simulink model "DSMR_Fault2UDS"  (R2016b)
settings: Solver=FixedStepDiscrete  StartTime=0.0  StopTime=10.0  FixedStep=0.02  RelTol=1e-3  EnableMultiTasking=on
undefined symbols (not defined in the file): bin2dec
libraries: simulink x312
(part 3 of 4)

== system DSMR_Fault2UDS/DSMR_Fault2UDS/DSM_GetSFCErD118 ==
  DFC : Inport  OutDataTypeStr=uint8
  DFC_IsoChkLv1_1 : simulink/Logic and Bit Operations/Bitwise Operator  logicop=AND  UseBitMask=on  BitMask=bin2dec('00011000')  BitMaskRealWorld=Stored Integer
  DFC_IsoChkLv1_1_compare : simulink/Logic and Bit Operations/Compare To Constant  relop===  const=24  OutDataTypeStr=boolean
  y : Outport
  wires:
  DFC_IsoChkLv1_1_compare/1 -> y/1
  DFC/1 -> DFC_IsoChkLv1_1/1
  DFC_IsoChkLv1_1/1 -> DFC_IsoChkLv1_1_compare/1

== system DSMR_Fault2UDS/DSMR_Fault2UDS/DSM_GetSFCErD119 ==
  DFC : Inport  OutDataTypeStr=uint8
  DFC_IsoChkLv1_1 : simulink/Logic and Bit Operations/Bitwise Operator  logicop=AND  UseBitMask=on  BitMask=bin2dec('00011000')  BitMaskRealWorld=Stored Integer
  DFC_IsoChkLv1_1_compare : simulink/Logic and Bit Operations/Compare To Constant  relop===  const=24  OutDataTypeStr=boolean
  y : Outport
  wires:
  DFC_IsoChkLv1_1_compare/1 -> y/1
  DFC/1 -> DFC_IsoChkLv1_1/1
  DFC_IsoChkLv1_1/1 -> DFC_IsoChkLv1_1_compare/1

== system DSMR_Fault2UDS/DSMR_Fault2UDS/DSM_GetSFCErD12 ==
  DFC : Inport  OutDataTypeStr=uint8
  DFC_IsoChkLv1_1 : simulink/Logic and Bit Operations/Bitwise Operator  logicop=AND  UseBitMask=on  BitMask=bin2dec('00011000')  BitMaskRealWorld=Stored Integer
  DFC_IsoChkLv1_1_compare : simulink/Logic and Bit Operations/Compare To Constant  relop===  const=24  OutDataTypeStr=boolean
  y : Outport
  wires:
  DFC_IsoChkLv1_1_compare/1 -> y/1
  DFC/1 -> DFC_IsoChkLv1_1/1
  DFC_IsoChkLv1_1/1 -> DFC_IsoChkLv1_1_compare/1

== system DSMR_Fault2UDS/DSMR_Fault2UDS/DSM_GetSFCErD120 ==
  DFC : Inport  OutDataTypeStr=uint8
  DFC_IsoChkLv1_1 : simulink/Logic and Bit Operations/Bitwise Operator  logicop=AND  UseBitMask=on  BitMask=bin2dec('00011000')  BitMaskRealWorld=Stored Integer
  DFC_IsoChkLv1_1_compare : simulink/Logic and Bit Operations/Compare To Constant  relop===  const=24  OutDataTypeStr=boolean
  y : Outport
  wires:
  DFC_IsoChkLv1_1_compare/1 -> y/1
  DFC/1 -> DFC_IsoChkLv1_1/1
  DFC_IsoChkLv1_1/1 -> DFC_IsoChkLv1_1_compare/1

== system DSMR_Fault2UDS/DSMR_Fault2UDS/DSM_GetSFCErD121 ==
  DFC : Inport  OutDataTypeStr=uint8
  DFC_IsoChkLv1_1 : simulink/Logic and Bit Operations/Bitwise Operator  logicop=AND  UseBitMask=on  BitMask=bin2dec('00011000')  BitMaskRealWorld=Stored Integer
  DFC_IsoChkLv1_1_compare : simulink/Logic and Bit Operations/Compare To Constant  relop===  const=24  OutDataTypeStr=boolean
  y : Outport
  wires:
  DFC_IsoChkLv1_1_compare/1 -> y/1
  DFC/1 -> DFC_IsoChkLv1_1/1
  DFC_IsoChkLv1_1/1 -> DFC_IsoChkLv1_1_compare/1

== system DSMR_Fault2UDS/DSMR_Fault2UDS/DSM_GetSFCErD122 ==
  DFC : Inport  OutDataTypeStr=uint8
  DFC_IsoChkLv1_1 : simulink/Logic and Bit Operations/Bitwise Operator  logicop=AND  UseBitMask=on  BitMask=bin2dec('00011000')  BitMaskRealWorld=Stored Integer
  DFC_IsoChkLv1_1_compare : simulink/Logic and Bit Operations/Compare To Constant  relop===  const=24  OutDataTypeStr=boolean
  y : Outport
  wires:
  DFC_IsoChkLv1_1_compare/1 -> y/1
  DFC/1 -> DFC_IsoChkLv1_1/1
  DFC_IsoChkLv1_1/1 -> DFC_IsoChkLv1_1_compare/1

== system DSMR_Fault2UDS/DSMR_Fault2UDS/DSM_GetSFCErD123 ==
  DFC : Inport  OutDataTypeStr=uint8
  DFC_IsoChkLv1_1 : simulink/Logic and Bit Operations/Bitwise Operator  logicop=AND  UseBitMask=on  BitMask=bin2dec('00011000')  BitMaskRealWorld=Stored Integer
  DFC_IsoChkLv1_1_compare : simulink/Logic and Bit Operations/Compare To Constant  relop===  const=24  OutDataTypeStr=boolean
  y : Outport
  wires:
  DFC_IsoChkLv1_1_compare/1 -> y/1
  DFC/1 -> DFC_IsoChkLv1_1/1
  DFC_IsoChkLv1_1/1 -> DFC_IsoChkLv1_1_compare/1

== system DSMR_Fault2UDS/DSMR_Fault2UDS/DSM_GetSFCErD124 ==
  DFC : Inport  OutDataTypeStr=uint8
  DFC_IsoChkLv1_1 : simulink/Logic and Bit Operations/Bitwise Operator  logicop=AND  UseBitMask=on  BitMask=bin2dec('00011000')  BitMaskRealWorld=Stored Integer
  DFC_IsoChkLv1_1_compare : simulink/Logic and Bit Operations/Compare To Constant  relop===  const=24  OutDataTypeStr=boolean
  y : Outport
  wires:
  DFC_IsoChkLv1_1_compare/1 -> y/1
  DFC/1 -> DFC_IsoChkLv1_1/1
  DFC_IsoChkLv1_1/1 -> DFC_IsoChkLv1_1_compare/1

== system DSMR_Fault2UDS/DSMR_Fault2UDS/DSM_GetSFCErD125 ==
  DFC : Inport  OutDataTypeStr=uint8
  DFC_IsoChkLv1_1 : simulink/Logic and Bit Operations/Bitwise Operator  logicop=AND  UseBitMask=on  BitMask=bin2dec('00011000')  BitMaskRealWorld=Stored Integer
  DFC_IsoChkLv1_1_compare : simulink/Logic and Bit Operations/Compare To Constant  relop===  const=24  OutDataTypeStr=boolean
  y : Outport
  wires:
  DFC_IsoChkLv1_1_compare/1 -> y/1
  DFC/1 -> DFC_IsoChkLv1_1/1
  DFC_IsoChkLv1_1/1 -> DFC_IsoChkLv1_1_compare/1

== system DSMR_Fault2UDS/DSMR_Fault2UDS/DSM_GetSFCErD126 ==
  DFC : Inport  OutDataTypeStr=uint8
  DFC_IsoChkLv1_1 : simulink/Logic and Bit Operations/Bitwise Operator  logicop=AND  UseBitMask=on  BitMask=bin2dec('00011000')  BitMaskRealWorld=Stored Integer
  DFC_IsoChkLv1_1_compare : simulink/Logic and Bit Operations/Compare To Constant  relop===  const=24  OutDataTypeStr=boolean
  y : Outport
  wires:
  DFC_IsoChkLv1_1_compare/1 -> y/1
  DFC/1 -> DFC_IsoChkLv1_1/1
  DFC_IsoChkLv1_1/1 -> DFC_IsoChkLv1_1_compare/1

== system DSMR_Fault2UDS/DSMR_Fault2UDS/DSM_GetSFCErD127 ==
  DFC : Inport  OutDataTypeStr=uint8
  DFC_IsoChkLv1_1 : simulink/Logic and Bit Operations/Bitwise Operator  logicop=AND  UseBitMask=on  BitMask=bin2dec('00011000')  BitMaskRealWorld=Stored Integer
  DFC_IsoChkLv1_1_compare : simulink/Logic and Bit Operations/Compare To Constant  relop===  const=24  OutDataTypeStr=boolean
  y : Outport
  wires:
  DFC_IsoChkLv1_1_compare/1 -> y/1
  DFC/1 -> DFC_IsoChkLv1_1/1
  DFC_IsoChkLv1_1/1 -> DFC_IsoChkLv1_1_compare/1

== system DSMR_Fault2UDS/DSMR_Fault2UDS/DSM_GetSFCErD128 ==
  DFC : Inport  OutDataTypeStr=uint8
  DFC_IsoChkLv1_1 : simulink/Logic and Bit Operations/Bitwise Operator  logicop=AND  UseBitMask=on  BitMask=bin2dec('00011000')  BitMaskRealWorld=Stored Integer
  DFC_IsoChkLv1_1_compare : simulink/Logic and Bit Operations/Compare To Constant  relop===  const=24  OutDataTypeStr=boolean
  y : Outport
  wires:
  DFC_IsoChkLv1_1_compare/1 -> y/1
  DFC/1 -> DFC_IsoChkLv1_1/1
  DFC_IsoChkLv1_1/1 -> DFC_IsoChkLv1_1_compare/1

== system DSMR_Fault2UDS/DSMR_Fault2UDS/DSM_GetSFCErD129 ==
  DFC : Inport  OutDataTypeStr=uint8
  DFC_IsoChkLv1_1 : simulink/Logic and Bit Operations/Bitwise Operator  logicop=AND  UseBitMask=on  BitMask=bin2dec('00011000')  BitMaskRealWorld=Stored Integer
  DFC_IsoChkLv1_1_compare : simulink/Logic and Bit Operations/Compare To Constant  relop===  const=24  OutDataTypeStr=boolean
  y : Outport
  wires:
  DFC_IsoChkLv1_1_compare/1 -> y/1
  DFC/1 -> DFC_IsoChkLv1_1/1
  DFC_IsoChkLv1_1/1 -> DFC_IsoChkLv1_1_compare/1

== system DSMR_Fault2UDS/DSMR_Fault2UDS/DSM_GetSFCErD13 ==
  DFC : Inport  OutDataTypeStr=uint8
  DFC_IsoChkLv1_1 : simulink/Logic and Bit Operations/Bitwise Operator  logicop=AND  UseBitMask=on  BitMask=bin2dec('00011000')  BitMaskRealWorld=Stored Integer
  DFC_IsoChkLv1_1_compare : simulink/Logic and Bit Operations/Compare To Constant  relop===  const=24  OutDataTypeStr=boolean
  y : Outport
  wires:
  DFC_IsoChkLv1_1_compare/1 -> y/1
  DFC/1 -> DFC_IsoChkLv1_1/1
  DFC_IsoChkLv1_1/1 -> DFC_IsoChkLv1_1_compare/1

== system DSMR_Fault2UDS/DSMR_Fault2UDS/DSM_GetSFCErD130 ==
  DFC : Inport  OutDataTypeStr=uint8
  DFC_IsoChkLv1_1 : simulink/Logic and Bit Operations/Bitwise Operator  logicop=AND  UseBitMask=on  BitMask=bin2dec('00011000')  BitMaskRealWorld=Stored Integer
  DFC_IsoChkLv1_1_compare : simulink/Logic and Bit Operations/Compare To Constant  relop===  const=24  OutDataTypeStr=boolean
  y : Outport
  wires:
  DFC_IsoChkLv1_1_compare/1 -> y/1
  DFC/1 -> DFC_IsoChkLv1_1/1
  DFC_IsoChkLv1_1/1 -> DFC_IsoChkLv1_1_compare/1

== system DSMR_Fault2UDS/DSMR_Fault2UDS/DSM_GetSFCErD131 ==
  DFC : Inport  OutDataTypeStr=uint8
  DFC_IsoChkLv1_1 : simulink/Logic and Bit Operations/Bitwise Operator  logicop=AND  UseBitMask=on  BitMask=bin2dec('00011000')  BitMaskRealWorld=Stored Integer
  DFC_IsoChkLv1_1_compare : simulink/Logic and Bit Operations/Compare To Constant  relop===  const=24  OutDataTypeStr=boolean
  y : Outport
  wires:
  DFC_IsoChkLv1_1_compare/1 -> y/1
  DFC/1 -> DFC_IsoChkLv1_1/1
  DFC_IsoChkLv1_1/1 -> DFC_IsoChkLv1_1_compare/1

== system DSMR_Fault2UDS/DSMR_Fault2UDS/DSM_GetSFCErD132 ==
  DFC : Inport  OutDataTypeStr=uint8
  DFC_IsoChkLv1_1 : simulink/Logic and Bit Operations/Bitwise Operator  logicop=AND  UseBitMask=on  BitMask=bin2dec('00011000')  BitMaskRealWorld=Stored Integer
  DFC_IsoChkLv1_1_compare : simulink/Logic and Bit Operations/Compare To Constant  relop===  const=24  OutDataTypeStr=boolean
  y : Outport
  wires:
  DFC_IsoChkLv1_1_compare/1 -> y/1
  DFC/1 -> DFC_IsoChkLv1_1/1
  DFC_IsoChkLv1_1/1 -> DFC_IsoChkLv1_1_compare/1

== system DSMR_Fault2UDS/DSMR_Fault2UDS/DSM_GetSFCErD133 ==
  DFC : Inport  OutDataTypeStr=uint8
  DFC_IsoChkLv1_1 : simulink/Logic and Bit Operations/Bitwise Operator  logicop=AND  UseBitMask=on  BitMask=bin2dec('00011000')  BitMaskRealWorld=Stored Integer
  DFC_IsoChkLv1_1_compare : simulink/Logic and Bit Operations/Compare To Constant  relop===  const=24  OutDataTypeStr=boolean
  y : Outport
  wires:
  DFC_IsoChkLv1_1_compare/1 -> y/1
  DFC/1 -> DFC_IsoChkLv1_1/1
  DFC_IsoChkLv1_1/1 -> DFC_IsoChkLv1_1_compare/1

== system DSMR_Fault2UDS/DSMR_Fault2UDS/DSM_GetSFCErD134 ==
  DFC : Inport  OutDataTypeStr=uint8
  DFC_IsoChkLv1_1 : simulink/Logic and Bit Operations/Bitwise Operator  logicop=AND  UseBitMask=on  BitMask=bin2dec('00011000')  BitMaskRealWorld=Stored Integer
  DFC_IsoChkLv1_1_compare : simulink/Logic and Bit Operations/Compare To Constant  relop===  const=24  OutDataTypeStr=boolean
  y : Outport
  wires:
  DFC_IsoChkLv1_1_compare/1 -> y/1
  DFC/1 -> DFC_IsoChkLv1_1/1
  DFC_IsoChkLv1_1/1 -> DFC_IsoChkLv1_1_compare/1

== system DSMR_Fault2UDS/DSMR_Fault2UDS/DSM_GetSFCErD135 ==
  DFC : Inport  OutDataTypeStr=uint8
  DFC_IsoChkLv1_1 : simulink/Logic and Bit Operations/Bitwise Operator  logicop=AND  UseBitMask=on  BitMask=bin2dec('00011000')  BitMaskRealWorld=Stored Integer
  DFC_IsoChkLv1_1_compare : simulink/Logic and Bit Operations/Compare To Constant  relop===  const=24  OutDataTypeStr=boolean
  y : Outport
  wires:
  DFC_IsoChkLv1_1_compare/1 -> y/1
  DFC/1 -> DFC_IsoChkLv1_1/1
  DFC_IsoChkLv1_1/1 -> DFC_IsoChkLv1_1_compare/1

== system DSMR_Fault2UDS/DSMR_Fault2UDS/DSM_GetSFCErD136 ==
  DFC : Inport  OutDataTypeStr=uint8
  DFC_IsoChkLv1_1 : simulink/Logic and Bit Operations/Bitwise Operator  logicop=AND  UseBitMask=on  BitMask=bin2dec('00011000')  BitMaskRealWorld=Stored Integer
  DFC_IsoChkLv1_1_compare : simulink/Logic and Bit Operations/Compare To Constant  relop===  const=24  OutDataTypeStr=boolean
  y : Outport
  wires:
  DFC_IsoChkLv1_1_compare/1 -> y/1
  DFC/1 -> DFC_IsoChkLv1_1/1
  DFC_IsoChkLv1_1/1 -> DFC_IsoChkLv1_1_compare/1

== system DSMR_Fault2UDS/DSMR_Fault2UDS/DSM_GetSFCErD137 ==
  DFC : Inport  OutDataTypeStr=uint8
  DFC_IsoChkLv1_1 : simulink/Logic and Bit Operations/Bitwise Operator  logicop=AND  UseBitMask=on  BitMask=bin2dec('00011000')  BitMaskRealWorld=Stored Integer
  DFC_IsoChkLv1_1_compare : simulink/Logic and Bit Operations/Compare To Constant  relop===  const=24  OutDataTypeStr=boolean
  y : Outport
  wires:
  DFC_IsoChkLv1_1_compare/1 -> y/1
  DFC/1 -> DFC_IsoChkLv1_1/1
  DFC_IsoChkLv1_1/1 -> DFC_IsoChkLv1_1_compare/1

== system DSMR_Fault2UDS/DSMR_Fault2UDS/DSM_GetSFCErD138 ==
  DFC : Inport  OutDataTypeStr=uint8
  DFC_IsoChkLv1_1 : simulink/Logic and Bit Operations/Bitwise Operator  logicop=AND  UseBitMask=on  BitMask=bin2dec('00011000')  BitMaskRealWorld=Stored Integer
  DFC_IsoChkLv1_1_compare : simulink/Logic and Bit Operations/Compare To Constant  relop===  const=24  OutDataTypeStr=boolean
  y : Outport
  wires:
  DFC_IsoChkLv1_1_compare/1 -> y/1
  DFC/1 -> DFC_IsoChkLv1_1/1
  DFC_IsoChkLv1_1/1 -> DFC_IsoChkLv1_1_compare/1

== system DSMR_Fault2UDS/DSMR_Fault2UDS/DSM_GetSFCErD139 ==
  DFC : Inport  OutDataTypeStr=uint8
  DFC_IsoChkLv1_1 : simulink/Logic and Bit Operations/Bitwise Operator  logicop=AND  UseBitMask=on  BitMask=bin2dec('00011000')  BitMaskRealWorld=Stored Integer
  DFC_IsoChkLv1_1_compare : simulink/Logic and Bit Operations/Compare To Constant  relop===  const=24  OutDataTypeStr=boolean
  y : Outport
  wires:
  DFC_IsoChkLv1_1_compare/1 -> y/1
  DFC/1 -> DFC_IsoChkLv1_1/1
  DFC_IsoChkLv1_1/1 -> DFC_IsoChkLv1_1_compare/1

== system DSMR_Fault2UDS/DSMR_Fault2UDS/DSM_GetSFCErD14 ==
  DFC : Inport  OutDataTypeStr=uint8
  DFC_IsoChkLv1_1 : simulink/Logic and Bit Operations/Bitwise Operator  logicop=AND  UseBitMask=on  BitMask=bin2dec('00011000')  BitMaskRealWorld=Stored Integer
  DFC_IsoChkLv1_1_compare : simulink/Logic and Bit Operations/Compare To Constant  relop===  const=24  OutDataTypeStr=boolean
  y : Outport
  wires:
  DFC_IsoChkLv1_1_compare/1 -> y/1
  DFC/1 -> DFC_IsoChkLv1_1/1
  DFC_IsoChkLv1_1/1 -> DFC_IsoChkLv1_1_compare/1

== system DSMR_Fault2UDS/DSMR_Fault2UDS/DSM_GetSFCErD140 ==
  DFC : Inport  OutDataTypeStr=uint8
  DFC_IsoChkLv1_1 : simulink/Logic and Bit Operations/Bitwise Operator  logicop=AND  UseBitMask=on  BitMask=bin2dec('00011000')  BitMaskRealWorld=Stored Integer
  DFC_IsoChkLv1_1_compare : simulink/Logic and Bit Operations/Compare To Constant  relop===  const=24  OutDataTypeStr=boolean
  y : Outport
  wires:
  DFC_IsoChkLv1_1_compare/1 -> y/1
  DFC/1 -> DFC_IsoChkLv1_1/1
  DFC_IsoChkLv1_1/1 -> DFC_IsoChkLv1_1_compare/1

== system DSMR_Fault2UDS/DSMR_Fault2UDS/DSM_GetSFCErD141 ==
  DFC : Inport  OutDataTypeStr=uint8
  DFC_IsoChkLv1_1 : simulink/Logic and Bit Operations/Bitwise Operator  logicop=AND  UseBitMask=on  BitMask=bin2dec('00011000')  BitMaskRealWorld=Stored Integer
  DFC_IsoChkLv1_1_compare : simulink/Logic and Bit Operations/Compare To Constant  relop===  const=24  OutDataTypeStr=boolean
  y : Outport
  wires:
  DFC_IsoChkLv1_1_compare/1 -> y/1
  DFC/1 -> DFC_IsoChkLv1_1/1
  DFC_IsoChkLv1_1/1 -> DFC_IsoChkLv1_1_compare/1

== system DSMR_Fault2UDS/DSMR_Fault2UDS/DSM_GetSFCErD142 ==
  DFC : Inport  OutDataTypeStr=uint8
  DFC_IsoChkLv1_1 : simulink/Logic and Bit Operations/Bitwise Operator  logicop=AND  UseBitMask=on  BitMask=bin2dec('00011000')  BitMaskRealWorld=Stored Integer
  DFC_IsoChkLv1_1_compare : simulink/Logic and Bit Operations/Compare To Constant  relop===  const=24  OutDataTypeStr=boolean
  y : Outport
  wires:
  DFC_IsoChkLv1_1_compare/1 -> y/1
  DFC/1 -> DFC_IsoChkLv1_1/1
  DFC_IsoChkLv1_1/1 -> DFC_IsoChkLv1_1_compare/1

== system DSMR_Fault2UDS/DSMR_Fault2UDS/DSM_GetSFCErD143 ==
  DFC : Inport  OutDataTypeStr=uint8
  DFC_IsoChkLv1_1 : simulink/Logic and Bit Operations/Bitwise Operator  logicop=AND  UseBitMask=on  BitMask=bin2dec('00011000')  BitMaskRealWorld=Stored Integer
  DFC_IsoChkLv1_1_compare : simulink/Logic and Bit Operations/Compare To Constant  relop===  const=24  OutDataTypeStr=boolean
  y : Outport
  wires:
  DFC_IsoChkLv1_1_compare/1 -> y/1
  DFC/1 -> DFC_IsoChkLv1_1/1
  DFC_IsoChkLv1_1/1 -> DFC_IsoChkLv1_1_compare/1

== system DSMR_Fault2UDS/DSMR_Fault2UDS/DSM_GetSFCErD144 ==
  DFC : Inport  OutDataTypeStr=uint8
  DFC_IsoChkLv1_1 : simulink/Logic and Bit Operations/Bitwise Operator  logicop=AND  UseBitMask=on  BitMask=bin2dec('00011000')  BitMaskRealWorld=Stored Integer
  DFC_IsoChkLv1_1_compare : simulink/Logic and Bit Operations/Compare To Constant  relop===  const=24  OutDataTypeStr=boolean
  y : Outport
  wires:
  DFC_IsoChkLv1_1_compare/1 -> y/1
  DFC/1 -> DFC_IsoChkLv1_1/1
  DFC_IsoChkLv1_1/1 -> DFC_IsoChkLv1_1_compare/1

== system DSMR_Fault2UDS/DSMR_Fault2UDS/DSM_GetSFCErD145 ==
  DFC : Inport  OutDataTypeStr=uint8
  DFC_IsoChkLv1_1 : simulink/Logic and Bit Operations/Bitwise Operator  logicop=AND  UseBitMask=on  BitMask=bin2dec('00011000')  BitMaskRealWorld=Stored Integer
  DFC_IsoChkLv1_1_compare : simulink/Logic and Bit Operations/Compare To Constant  relop===  const=24  OutDataTypeStr=boolean
  y : Outport
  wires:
  DFC_IsoChkLv1_1_compare/1 -> y/1
  DFC/1 -> DFC_IsoChkLv1_1/1
  DFC_IsoChkLv1_1/1 -> DFC_IsoChkLv1_1_compare/1

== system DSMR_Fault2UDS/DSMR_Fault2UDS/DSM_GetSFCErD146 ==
  DFC : Inport  OutDataTypeStr=uint8
  DFC_IsoChkLv1_1 : simulink/Logic and Bit Operations/Bitwise Operator  logicop=AND  UseBitMask=on  BitMask=bin2dec('00011000')  BitMaskRealWorld=Stored Integer
  DFC_IsoChkLv1_1_compare : simulink/Logic and Bit Operations/Compare To Constant  relop===  const=24  OutDataTypeStr=boolean
  y : Outport
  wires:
  DFC_IsoChkLv1_1_compare/1 -> y/1
  DFC/1 -> DFC_IsoChkLv1_1/1
  DFC_IsoChkLv1_1/1 -> DFC_IsoChkLv1_1_compare/1

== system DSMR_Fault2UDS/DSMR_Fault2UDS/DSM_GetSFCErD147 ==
  DFC : Inport  OutDataTypeStr=uint8
  DFC_IsoChkLv1_1 : simulink/Logic and Bit Operations/Bitwise Operator  logicop=AND  UseBitMask=on  BitMask=bin2dec('00011000')  BitMaskRealWorld=Stored Integer
  DFC_IsoChkLv1_1_compare : simulink/Logic and Bit Operations/Compare To Constant  relop===  const=24  OutDataTypeStr=boolean
  y : Outport
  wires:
  DFC_IsoChkLv1_1_compare/1 -> y/1
  DFC/1 -> DFC_IsoChkLv1_1/1
  DFC_IsoChkLv1_1/1 -> DFC_IsoChkLv1_1_compare/1

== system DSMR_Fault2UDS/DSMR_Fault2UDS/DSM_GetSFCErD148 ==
  DFC : Inport  OutDataTypeStr=uint8
  DFC_IsoChkLv1_1 : simulink/Logic and Bit Operations/Bitwise Operator  logicop=AND  UseBitMask=on  BitMask=bin2dec('00011000')  BitMaskRealWorld=Stored Integer
  DFC_IsoChkLv1_1_compare : simulink/Logic and Bit Operations/Compare To Constant  relop===  const=24  OutDataTypeStr=boolean
  y : Outport
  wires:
  DFC_IsoChkLv1_1_compare/1 -> y/1
  DFC/1 -> DFC_IsoChkLv1_1/1
  DFC_IsoChkLv1_1/1 -> DFC_IsoChkLv1_1_compare/1

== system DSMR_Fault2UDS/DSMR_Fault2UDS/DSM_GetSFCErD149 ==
  DFC : Inport  OutDataTypeStr=uint8
  DFC_IsoChkLv1_1 : simulink/Logic and Bit Operations/Bitwise Operator  logicop=AND  UseBitMask=on  BitMask=bin2dec('00011000')  BitMaskRealWorld=Stored Integer
  DFC_IsoChkLv1_1_compare : simulink/Logic and Bit Operations/Compare To Constant  relop===  const=24  OutDataTypeStr=boolean
  y : Outport
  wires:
  DFC_IsoChkLv1_1_compare/1 -> y/1
  DFC/1 -> DFC_IsoChkLv1_1/1
  DFC_IsoChkLv1_1/1 -> DFC_IsoChkLv1_1_compare/1

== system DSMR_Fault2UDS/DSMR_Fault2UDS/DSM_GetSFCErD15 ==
  DFC : Inport  OutDataTypeStr=uint8
  DFC_IsoChkLv1_1 : simulink/Logic and Bit Operations/Bitwise Operator  logicop=AND  UseBitMask=on  BitMask=bin2dec('00011000')  BitMaskRealWorld=Stored Integer
  DFC_IsoChkLv1_1_compare : simulink/Logic and Bit Operations/Compare To Constant  relop===  const=24  OutDataTypeStr=boolean
  y : Outport
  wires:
  DFC_IsoChkLv1_1_compare/1 -> y/1
  DFC/1 -> DFC_IsoChkLv1_1/1
  DFC_IsoChkLv1_1/1 -> DFC_IsoChkLv1_1_compare/1

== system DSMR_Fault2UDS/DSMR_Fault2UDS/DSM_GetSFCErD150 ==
  DFC : Inport  OutDataTypeStr=uint8
  DFC_IsoChkLv1_1 : simulink/Logic and Bit Operations/Bitwise Operator  logicop=AND  UseBitMask=on  BitMask=bin2dec('00011000')  BitMaskRealWorld=Stored Integer
  DFC_IsoChkLv1_1_compare : simulink/Logic and Bit Operations/Compare To Constant  relop===  const=24  OutDataTypeStr=boolean
  y : Outport
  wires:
  DFC_IsoChkLv1_1_compare/1 -> y/1
  DFC/1 -> DFC_IsoChkLv1_1/1
  DFC_IsoChkLv1_1/1 -> DFC_IsoChkLv1_1_compare/1

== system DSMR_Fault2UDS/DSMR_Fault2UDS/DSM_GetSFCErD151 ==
  DFC : Inport  OutDataTypeStr=uint8
  DFC_IsoChkLv1_1 : simulink/Logic and Bit Operations/Bitwise Operator  logicop=AND  UseBitMask=on  BitMask=bin2dec('00011000')  BitMaskRealWorld=Stored Integer
  DFC_IsoChkLv1_1_compare : simulink/Logic and Bit Operations/Compare To Constant  relop===  const=24  OutDataTypeStr=boolean
  y : Outport
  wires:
  DFC_IsoChkLv1_1_compare/1 -> y/1
  DFC/1 -> DFC_IsoChkLv1_1/1
  DFC_IsoChkLv1_1/1 -> DFC_IsoChkLv1_1_compare/1

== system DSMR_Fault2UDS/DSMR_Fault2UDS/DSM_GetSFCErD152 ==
  DFC : Inport  OutDataTypeStr=uint8
  DFC_IsoChkLv1_1 : simulink/Logic and Bit Operations/Bitwise Operator  logicop=AND  UseBitMask=on  BitMask=bin2dec('00011000')  BitMaskRealWorld=Stored Integer
  DFC_IsoChkLv1_1_compare : simulink/Logic and Bit Operations/Compare To Constant  relop===  const=24  OutDataTypeStr=boolean
  y : Outport
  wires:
  DFC_IsoChkLv1_1_compare/1 -> y/1
  DFC/1 -> DFC_IsoChkLv1_1/1
  DFC_IsoChkLv1_1/1 -> DFC_IsoChkLv1_1_compare/1

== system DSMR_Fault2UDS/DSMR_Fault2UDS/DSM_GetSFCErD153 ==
  DFC : Inport  OutDataTypeStr=uint8
  DFC_IsoChkLv1_1 : simulink/Logic and Bit Operations/Bitwise Operator  logicop=AND  UseBitMask=on  BitMask=bin2dec('00011000')  BitMaskRealWorld=Stored Integer
  DFC_IsoChkLv1_1_compare : simulink/Logic and Bit Operations/Compare To Constant  relop===  const=24  OutDataTypeStr=boolean
  y : Outport
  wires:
  DFC_IsoChkLv1_1_compare/1 -> y/1
  DFC/1 -> DFC_IsoChkLv1_1/1
  DFC_IsoChkLv1_1/1 -> DFC_IsoChkLv1_1_compare/1

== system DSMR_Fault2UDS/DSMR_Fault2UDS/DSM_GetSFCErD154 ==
  DFC : Inport  OutDataTypeStr=uint8
  DFC_IsoChkLv1_1 : simulink/Logic and Bit Operations/Bitwise Operator  logicop=AND  UseBitMask=on  BitMask=bin2dec('00011000')  BitMaskRealWorld=Stored Integer
  DFC_IsoChkLv1_1_compare : simulink/Logic and Bit Operations/Compare To Constant  relop===  const=24  OutDataTypeStr=boolean
  y : Outport
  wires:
  DFC_IsoChkLv1_1_compare/1 -> y/1
  DFC/1 -> DFC_IsoChkLv1_1/1
  DFC_IsoChkLv1_1/1 -> DFC_IsoChkLv1_1_compare/1

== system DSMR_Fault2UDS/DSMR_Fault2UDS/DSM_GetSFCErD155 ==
  DFC : Inport  OutDataTypeStr=uint8
  DFC_IsoChkLv1_1 : simulink/Logic and Bit Operations/Bitwise Operator  logicop=AND  UseBitMask=on  BitMask=bin2dec('00011000')  BitMaskRealWorld=Stored Integer
  DFC_IsoChkLv1_1_compare : simulink/Logic and Bit Operations/Compare To Constant  relop===  const=24  OutDataTypeStr=boolean
  y : Outport
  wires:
  DFC_IsoChkLv1_1_compare/1 -> y/1
  DFC/1 -> DFC_IsoChkLv1_1/1
  DFC_IsoChkLv1_1/1 -> DFC_IsoChkLv1_1_compare/1

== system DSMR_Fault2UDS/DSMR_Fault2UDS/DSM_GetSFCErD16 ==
  DFC : Inport  OutDataTypeStr=uint8
  DFC_IsoChkLv1_1 : simulink/Logic and Bit Operations/Bitwise Operator  logicop=AND  UseBitMask=on  BitMask=bin2dec('00011000')  BitMaskRealWorld=Stored Integer
  DFC_IsoChkLv1_1_compare : simulink/Logic and Bit Operations/Compare To Constant  relop===  const=24  OutDataTypeStr=boolean
  y : Outport
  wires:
  DFC_IsoChkLv1_1_compare/1 -> y/1
  DFC/1 -> DFC_IsoChkLv1_1/1
  DFC_IsoChkLv1_1/1 -> DFC_IsoChkLv1_1_compare/1

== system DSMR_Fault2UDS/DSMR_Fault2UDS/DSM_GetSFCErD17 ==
  DFC : Inport  OutDataTypeStr=uint8
  DFC_IsoChkLv1_1 : simulink/Logic and Bit Operations/Bitwise Operator  logicop=AND  UseBitMask=on  BitMask=bin2dec('00011000')  BitMaskRealWorld=Stored Integer
  DFC_IsoChkLv1_1_compare : simulink/Logic and Bit Operations/Compare To Constant  relop===  const=24  OutDataTypeStr=boolean
  y : Outport
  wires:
  DFC_IsoChkLv1_1_compare/1 -> y/1
  DFC/1 -> DFC_IsoChkLv1_1/1
  DFC_IsoChkLv1_1/1 -> DFC_IsoChkLv1_1_compare/1

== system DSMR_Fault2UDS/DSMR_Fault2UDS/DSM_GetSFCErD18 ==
  DFC : Inport  OutDataTypeStr=uint8
  DFC_IsoChkLv1_1 : simulink/Logic and Bit Operations/Bitwise Operator  logicop=AND  UseBitMask=on  BitMask=bin2dec('00011000')  BitMaskRealWorld=Stored Integer
  DFC_IsoChkLv1_1_compare : simulink/Logic and Bit Operations/Compare To Constant  relop===  const=24  OutDataTypeStr=boolean
  y : Outport
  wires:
  DFC_IsoChkLv1_1_compare/1 -> y/1
  DFC/1 -> DFC_IsoChkLv1_1/1
  DFC_IsoChkLv1_1/1 -> DFC_IsoChkLv1_1_compare/1

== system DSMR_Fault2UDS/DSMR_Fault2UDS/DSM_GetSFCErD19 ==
  DFC : Inport  OutDataTypeStr=uint8
  DFC_IsoChkLv1_1 : simulink/Logic and Bit Operations/Bitwise Operator  logicop=AND  UseBitMask=on  BitMask=bin2dec('00011000')  BitMaskRealWorld=Stored Integer
  DFC_IsoChkLv1_1_compare : simulink/Logic and Bit Operations/Compare To Constant  relop===  const=24  OutDataTypeStr=boolean
  y : Outport
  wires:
  DFC_IsoChkLv1_1_compare/1 -> y/1
  DFC/1 -> DFC_IsoChkLv1_1/1
  DFC_IsoChkLv1_1/1 -> DFC_IsoChkLv1_1_compare/1

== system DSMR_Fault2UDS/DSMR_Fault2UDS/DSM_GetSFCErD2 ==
  DFC : Inport  OutDataTypeStr=uint8
  DFC_IsoChkLv1_1 : simulink/Logic and Bit Operations/Bitwise Operator  logicop=AND  UseBitMask=on  BitMask=bin2dec('00011000')  BitMaskRealWorld=Stored Integer
  DFC_IsoChkLv1_1_compare : simulink/Logic and Bit Operations/Compare To Constant  relop===  const=24  OutDataTypeStr=boolean
  y : Outport
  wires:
  DFC_IsoChkLv1_1_compare/1 -> y/1
  DFC/1 -> DFC_IsoChkLv1_1/1
  DFC_IsoChkLv1_1/1 -> DFC_IsoChkLv1_1_compare/1

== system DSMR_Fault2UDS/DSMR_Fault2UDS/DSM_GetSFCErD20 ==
  DFC : Inport  OutDataTypeStr=uint8
  DFC_IsoChkLv1_1 : simulink/Logic and Bit Operations/Bitwise Operator  logicop=AND  UseBitMask=on  BitMask=bin2dec('00011000')  BitMaskRealWorld=Stored Integer
  DFC_IsoChkLv1_1_compare : simulink/Logic and Bit Operations/Compare To Constant  relop===  const=24  OutDataTypeStr=boolean
  y : Outport
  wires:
  DFC_IsoChkLv1_1_compare/1 -> y/1
  DFC/1 -> DFC_IsoChkLv1_1/1
  DFC_IsoChkLv1_1/1 -> DFC_IsoChkLv1_1_compare/1

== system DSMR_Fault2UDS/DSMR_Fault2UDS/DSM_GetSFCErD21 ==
  DFC : Inport  OutDataTypeStr=uint8
  DFC_IsoChkLv1_1 : simulink/Logic and Bit Operations/Bitwise Operator  logicop=AND  UseBitMask=on  BitMask=bin2dec('00011000')  BitMaskRealWorld=Stored Integer
  DFC_IsoChkLv1_1_compare : simulink/Logic and Bit Operations/Compare To Constant  relop===  const=24  OutDataTypeStr=boolean
  y : Outport
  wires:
  DFC_IsoChkLv1_1_compare/1 -> y/1
  DFC/1 -> DFC_IsoChkLv1_1/1
  DFC_IsoChkLv1_1/1 -> DFC_IsoChkLv1_1_compare/1

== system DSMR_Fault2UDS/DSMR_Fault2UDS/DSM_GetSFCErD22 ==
  DFC : Inport  OutDataTypeStr=uint8
  DFC_IsoChkLv1_1 : simulink/Logic and Bit Operations/Bitwise Operator  logicop=AND  UseBitMask=on  BitMask=bin2dec('00011000')  BitMaskRealWorld=Stored Integer
  DFC_IsoChkLv1_1_compare : simulink/Logic and Bit Operations/Compare To Constant  relop===  const=24  OutDataTypeStr=boolean
  y : Outport
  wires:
  DFC_IsoChkLv1_1_compare/1 -> y/1
  DFC/1 -> DFC_IsoChkLv1_1/1
  DFC_IsoChkLv1_1/1 -> DFC_IsoChkLv1_1_compare/1

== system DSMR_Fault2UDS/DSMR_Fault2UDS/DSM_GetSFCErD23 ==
  DFC : Inport  OutDataTypeStr=uint8
  DFC_IsoChkLv1_1 : simulink/Logic and Bit Operations/Bitwise Operator  logicop=AND  UseBitMask=on  BitMask=bin2dec('00011000')  BitMaskRealWorld=Stored Integer
  DFC_IsoChkLv1_1_compare : simulink/Logic and Bit Operations/Compare To Constant  relop===  const=24  OutDataTypeStr=boolean
  y : Outport
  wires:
  DFC_IsoChkLv1_1_compare/1 -> y/1
  DFC/1 -> DFC_IsoChkLv1_1/1
  DFC_IsoChkLv1_1/1 -> DFC_IsoChkLv1_1_compare/1

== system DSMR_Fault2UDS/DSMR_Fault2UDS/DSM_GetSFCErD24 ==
  DFC : Inport  OutDataTypeStr=uint8
  DFC_IsoChkLv1_1 : simulink/Logic and Bit Operations/Bitwise Operator  logicop=AND  UseBitMask=on  BitMask=bin2dec('00011000')  BitMaskRealWorld=Stored Integer
  DFC_IsoChkLv1_1_compare : simulink/Logic and Bit Operations/Compare To Constant  relop===  const=24  OutDataTypeStr=boolean
  y : Outport
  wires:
  DFC_IsoChkLv1_1_compare/1 -> y/1
  DFC/1 -> DFC_IsoChkLv1_1/1
  DFC_IsoChkLv1_1/1 -> DFC_IsoChkLv1_1_compare/1

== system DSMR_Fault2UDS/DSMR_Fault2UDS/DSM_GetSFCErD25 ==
  DFC : Inport  OutDataTypeStr=uint8
  DFC_IsoChkLv1_1 : simulink/Logic and Bit Operations/Bitwise Operator  logicop=AND  UseBitMask=on  BitMask=bin2dec('00011000')  BitMaskRealWorld=Stored Integer
  DFC_IsoChkLv1_1_compare : simulink/Logic and Bit Operations/Compare To Constant  relop===  const=24  OutDataTypeStr=boolean
  y : Outport
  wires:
  DFC_IsoChkLv1_1_compare/1 -> y/1
  DFC/1 -> DFC_IsoChkLv1_1/1
  DFC_IsoChkLv1_1/1 -> DFC_IsoChkLv1_1_compare/1

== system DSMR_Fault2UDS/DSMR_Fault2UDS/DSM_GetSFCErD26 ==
  DFC : Inport  OutDataTypeStr=uint8
  DFC_IsoChkLv1_1 : simulink/Logic and Bit Operations/Bitwise Operator  logicop=AND  UseBitMask=on  BitMask=bin2dec('00011000')  BitMaskRealWorld=Stored Integer
  DFC_IsoChkLv1_1_compare : simulink/Logic and Bit Operations/Compare To Constant  relop===  const=24  OutDataTypeStr=boolean
  y : Outport
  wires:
  DFC_IsoChkLv1_1_compare/1 -> y/1
  DFC/1 -> DFC_IsoChkLv1_1/1
  DFC_IsoChkLv1_1/1 -> DFC_IsoChkLv1_1_compare/1

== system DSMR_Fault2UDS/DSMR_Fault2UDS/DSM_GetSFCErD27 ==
  DFC : Inport  OutDataTypeStr=uint8
  DFC_IsoChkLv1_1 : simulink/Logic and Bit Operations/Bitwise Operator  logicop=AND  UseBitMask=on  BitMask=bin2dec('00011000')  BitMaskRealWorld=Stored Integer
  DFC_IsoChkLv1_1_compare : simulink/Logic and Bit Operations/Compare To Constant  relop===  const=24  OutDataTypeStr=boolean
  y : Outport
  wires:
  DFC_IsoChkLv1_1_compare/1 -> y/1
  DFC/1 -> DFC_IsoChkLv1_1/1
  DFC_IsoChkLv1_1/1 -> DFC_IsoChkLv1_1_compare/1

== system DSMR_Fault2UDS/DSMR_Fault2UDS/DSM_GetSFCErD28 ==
  DFC : Inport  OutDataTypeStr=uint8
  DFC_IsoChkLv1_1 : simulink/Logic and Bit Operations/Bitwise Operator  logicop=AND  UseBitMask=on  BitMask=bin2dec('00011000')  BitMaskRealWorld=Stored Integer
  DFC_IsoChkLv1_1_compare : simulink/Logic and Bit Operations/Compare To Constant  relop===  const=24  OutDataTypeStr=boolean
  y : Outport
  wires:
  DFC_IsoChkLv1_1_compare/1 -> y/1
  DFC/1 -> DFC_IsoChkLv1_1/1
  DFC_IsoChkLv1_1/1 -> DFC_IsoChkLv1_1_compare/1

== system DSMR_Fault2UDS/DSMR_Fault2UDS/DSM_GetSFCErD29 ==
  DFC : Inport  OutDataTypeStr=uint8
  DFC_IsoChkLv1_1 : simulink/Logic and Bit Operations/Bitwise Operator  logicop=AND  UseBitMask=on  BitMask=bin2dec('00011000')  BitMaskRealWorld=Stored Integer
  DFC_IsoChkLv1_1_compare : simulink/Logic and Bit Operations/Compare To Constant  relop===  const=24  OutDataTypeStr=boolean
  y : Outport
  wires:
  DFC_IsoChkLv1_1_compare/1 -> y/1
  DFC/1 -> DFC_IsoChkLv1_1/1
  DFC_IsoChkLv1_1/1 -> DFC_IsoChkLv1_1_compare/1

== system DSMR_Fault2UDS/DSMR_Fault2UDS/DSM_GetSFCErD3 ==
  DFC : Inport  OutDataTypeStr=uint8
  DFC_IsoChkLv1_1 : simulink/Logic and Bit Operations/Bitwise Operator  logicop=AND  UseBitMask=on  BitMask=bin2dec('00011000')  BitMaskRealWorld=Stored Integer
  DFC_IsoChkLv1_1_compare : simulink/Logic and Bit Operations/Compare To Constant  relop===  const=24  OutDataTypeStr=boolean
  y : Outport
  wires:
  DFC_IsoChkLv1_1_compare/1 -> y/1
  DFC/1 -> DFC_IsoChkLv1_1/1
  DFC_IsoChkLv1_1/1 -> DFC_IsoChkLv1_1_compare/1

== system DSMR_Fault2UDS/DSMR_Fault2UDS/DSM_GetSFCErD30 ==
  DFC : Inport  OutDataTypeStr=uint8
  DFC_IsoChkLv1_1 : simulink/Logic and Bit Operations/Bitwise Operator  logicop=AND  UseBitMask=on  BitMask=bin2dec('00011000')  BitMaskRealWorld=Stored Integer
  DFC_IsoChkLv1_1_compare : simulink/Logic and Bit Operations/Compare To Constant  relop===  const=24  OutDataTypeStr=boolean
  y : Outport
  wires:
  DFC_IsoChkLv1_1_compare/1 -> y/1
  DFC/1 -> DFC_IsoChkLv1_1/1
  DFC_IsoChkLv1_1/1 -> DFC_IsoChkLv1_1_compare/1

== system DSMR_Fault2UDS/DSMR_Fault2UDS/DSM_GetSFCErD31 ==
  DFC : Inport  OutDataTypeStr=uint8
  DFC_IsoChkLv1_1 : simulink/Logic and Bit Operations/Bitwise Operator  logicop=AND  UseBitMask=on  BitMask=bin2dec('00011000')  BitMaskRealWorld=Stored Integer
  DFC_IsoChkLv1_1_compare : simulink/Logic and Bit Operations/Compare To Constant  relop===  const=24  OutDataTypeStr=boolean
  y : Outport
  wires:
  DFC_IsoChkLv1_1_compare/1 -> y/1
  DFC/1 -> DFC_IsoChkLv1_1/1
  DFC_IsoChkLv1_1/1 -> DFC_IsoChkLv1_1_compare/1

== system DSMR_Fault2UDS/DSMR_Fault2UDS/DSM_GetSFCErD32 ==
  DFC : Inport  OutDataTypeStr=uint8
  DFC_IsoChkLv1_1 : simulink/Logic and Bit Operations/Bitwise Operator  logicop=AND  UseBitMask=on  BitMask=bin2dec('00011000')  BitMaskRealWorld=Stored Integer
  DFC_IsoChkLv1_1_compare : simulink/Logic and Bit Operations/Compare To Constant  relop===  const=24  OutDataTypeStr=boolean
  y : Outport
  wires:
  DFC_IsoChkLv1_1_compare/1 -> y/1
  DFC/1 -> DFC_IsoChkLv1_1/1
  DFC_IsoChkLv1_1/1 -> DFC_IsoChkLv1_1_compare/1

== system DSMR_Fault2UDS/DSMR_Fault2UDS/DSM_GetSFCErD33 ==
  DFC : Inport  OutDataTypeStr=uint8
  DFC_IsoChkLv1_1 : simulink/Logic and Bit Operations/Bitwise Operator  logicop=AND  UseBitMask=on  BitMask=bin2dec('00011000')  BitMaskRealWorld=Stored Integer
  DFC_IsoChkLv1_1_compare : simulink/Logic and Bit Operations/Compare To Constant  relop===  const=24  OutDataTypeStr=boolean
  y : Outport
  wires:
  DFC_IsoChkLv1_1_compare/1 -> y/1
  DFC/1 -> DFC_IsoChkLv1_1/1
  DFC_IsoChkLv1_1/1 -> DFC_IsoChkLv1_1_compare/1

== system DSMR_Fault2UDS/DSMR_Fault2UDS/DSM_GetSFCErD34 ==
  DFC : Inport  OutDataTypeStr=uint8
  DFC_IsoChkLv1_1 : simulink/Logic and Bit Operations/Bitwise Operator  logicop=AND  UseBitMask=on  BitMask=bin2dec('00011000')  BitMaskRealWorld=Stored Integer
  DFC_IsoChkLv1_1_compare : simulink/Logic and Bit Operations/Compare To Constant  relop===  const=24  OutDataTypeStr=boolean
  y : Outport
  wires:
  DFC_IsoChkLv1_1_compare/1 -> y/1
  DFC/1 -> DFC_IsoChkLv1_1/1
  DFC_IsoChkLv1_1/1 -> DFC_IsoChkLv1_1_compare/1

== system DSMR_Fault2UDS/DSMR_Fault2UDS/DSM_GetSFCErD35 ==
  DFC : Inport  OutDataTypeStr=uint8
  DFC_IsoChkLv1_1 : simulink/Logic and Bit Operations/Bitwise Operator  logicop=AND  UseBitMask=on  BitMask=bin2dec('00011000')  BitMaskRealWorld=Stored Integer
  DFC_IsoChkLv1_1_compare : simulink/Logic and Bit Operations/Compare To Constant  relop===  const=24  OutDataTypeStr=boolean
  y : Outport
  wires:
  DFC_IsoChkLv1_1_compare/1 -> y/1
  DFC/1 -> DFC_IsoChkLv1_1/1
  DFC_IsoChkLv1_1/1 -> DFC_IsoChkLv1_1_compare/1

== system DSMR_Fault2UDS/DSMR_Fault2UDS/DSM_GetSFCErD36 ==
  DFC : Inport  OutDataTypeStr=uint8
  DFC_IsoChkLv1_1 : simulink/Logic and Bit Operations/Bitwise Operator  logicop=AND  UseBitMask=on  BitMask=bin2dec('00011000')  BitMaskRealWorld=Stored Integer
  DFC_IsoChkLv1_1_compare : simulink/Logic and Bit Operations/Compare To Constant  relop===  const=24  OutDataTypeStr=boolean
  y : Outport
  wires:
  DFC_IsoChkLv1_1_compare/1 -> y/1
  DFC/1 -> DFC_IsoChkLv1_1/1
  DFC_IsoChkLv1_1/1 -> DFC_IsoChkLv1_1_compare/1

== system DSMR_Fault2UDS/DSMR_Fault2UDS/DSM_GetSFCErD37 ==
  DFC : Inport  OutDataTypeStr=uint8
  DFC_IsoChkLv1_1 : simulink/Logic and Bit Operations/Bitwise Operator  logicop=AND  UseBitMask=on  BitMask=bin2dec('00011000')  BitMaskRealWorld=Stored Integer
  DFC_IsoChkLv1_1_compare : simulink/Logic and Bit Operations/Compare To Constant  relop===  const=24  OutDataTypeStr=boolean
  y : Outport
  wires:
  DFC_IsoChkLv1_1_compare/1 -> y/1
  DFC/1 -> DFC_IsoChkLv1_1/1
  DFC_IsoChkLv1_1/1 -> DFC_IsoChkLv1_1_compare/1

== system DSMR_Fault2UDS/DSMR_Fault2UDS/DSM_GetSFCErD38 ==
  DFC : Inport  OutDataTypeStr=uint8
  DFC_IsoChkLv1_1 : simulink/Logic and Bit Operations/Bitwise Operator  logicop=AND  UseBitMask=on  BitMask=bin2dec('00011000')  BitMaskRealWorld=Stored Integer
  DFC_IsoChkLv1_1_compare : simulink/Logic and Bit Operations/Compare To Constant  relop===  const=24  OutDataTypeStr=boolean
  y : Outport
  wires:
  DFC_IsoChkLv1_1_compare/1 -> y/1
  DFC/1 -> DFC_IsoChkLv1_1/1
  DFC_IsoChkLv1_1/1 -> DFC_IsoChkLv1_1_compare/1

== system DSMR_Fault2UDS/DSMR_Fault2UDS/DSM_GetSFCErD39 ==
  DFC : Inport  OutDataTypeStr=uint8
  DFC_IsoChkLv1_1 : simulink/Logic and Bit Operations/Bitwise Operator  logicop=AND  UseBitMask=on  BitMask=bin2dec('00011000')  BitMaskRealWorld=Stored Integer
  DFC_IsoChkLv1_1_compare : simulink/Logic and Bit Operations/Compare To Constant  relop===  const=24  OutDataTypeStr=boolean
  y : Outport
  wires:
  DFC_IsoChkLv1_1_compare/1 -> y/1
  DFC/1 -> DFC_IsoChkLv1_1/1
  DFC_IsoChkLv1_1/1 -> DFC_IsoChkLv1_1_compare/1

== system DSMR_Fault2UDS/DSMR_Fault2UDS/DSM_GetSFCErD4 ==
  DFC : Inport  OutDataTypeStr=uint8
  DFC_IsoChkLv1_1 : simulink/Logic and Bit Operations/Bitwise Operator  logicop=AND  UseBitMask=on  BitMask=bin2dec('00011000')  BitMaskRealWorld=Stored Integer
  DFC_IsoChkLv1_1_compare : simulink/Logic and Bit Operations/Compare To Constant  relop===  const=24  OutDataTypeStr=boolean
  y : Outport
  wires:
  DFC_IsoChkLv1_1_compare/1 -> y/1
  DFC/1 -> DFC_IsoChkLv1_1/1
  DFC_IsoChkLv1_1/1 -> DFC_IsoChkLv1_1_compare/1

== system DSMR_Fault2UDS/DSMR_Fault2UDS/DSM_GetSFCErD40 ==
  DFC : Inport  OutDataTypeStr=uint8
  DFC_IsoChkLv1_1 : simulink/Logic and Bit Operations/Bitwise Operator  logicop=AND  UseBitMask=on  BitMask=bin2dec('00011000')  BitMaskRealWorld=Stored Integer
  DFC_IsoChkLv1_1_compare : simulink/Logic and Bit Operations/Compare To Constant  relop===  const=24  OutDataTypeStr=boolean
  y : Outport
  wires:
  DFC_IsoChkLv1_1_compare/1 -> y/1
  DFC/1 -> DFC_IsoChkLv1_1/1
  DFC_IsoChkLv1_1/1 -> DFC_IsoChkLv1_1_compare/1

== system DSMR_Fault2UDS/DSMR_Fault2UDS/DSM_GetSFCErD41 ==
  DFC : Inport  OutDataTypeStr=uint8
  DFC_IsoChkLv1_1 : simulink/Logic and Bit Operations/Bitwise Operator  logicop=AND  UseBitMask=on  BitMask=bin2dec('00011000')  BitMaskRealWorld=Stored Integer
  DFC_IsoChkLv1_1_compare : simulink/Logic and Bit Operations/Compare To Constant  relop===  const=24  OutDataTypeStr=boolean
  y : Outport
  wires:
  DFC_IsoChkLv1_1_compare/1 -> y/1
  DFC/1 -> DFC_IsoChkLv1_1/1
  DFC_IsoChkLv1_1/1 -> DFC_IsoChkLv1_1_compare/1

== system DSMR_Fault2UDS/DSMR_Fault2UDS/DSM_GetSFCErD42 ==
  DFC : Inport  OutDataTypeStr=uint8
  DFC_IsoChkLv1_1 : simulink/Logic and Bit Operations/Bitwise Operator  logicop=AND  UseBitMask=on  BitMask=bin2dec('00011000')  BitMaskRealWorld=Stored Integer
  DFC_IsoChkLv1_1_compare : simulink/Logic and Bit Operations/Compare To Constant  relop===  const=24  OutDataTypeStr=boolean
  y : Outport
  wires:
  DFC_IsoChkLv1_1_compare/1 -> y/1
  DFC/1 -> DFC_IsoChkLv1_1/1
  DFC_IsoChkLv1_1/1 -> DFC_IsoChkLv1_1_compare/1

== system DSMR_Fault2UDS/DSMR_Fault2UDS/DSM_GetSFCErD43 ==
  DFC : Inport  OutDataTypeStr=uint8
  DFC_IsoChkLv1_1 : simulink/Logic and Bit Operations/Bitwise Operator  logicop=AND  UseBitMask=on  BitMask=bin2dec('00011000')  BitMaskRealWorld=Stored Integer
  DFC_IsoChkLv1_1_compare : simulink/Logic and Bit Operations/Compare To Constant  relop===  const=24  OutDataTypeStr=boolean
  y : Outport
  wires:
  DFC_IsoChkLv1_1_compare/1 -> y/1
  DFC/1 -> DFC_IsoChkLv1_1/1
  DFC_IsoChkLv1_1/1 -> DFC_IsoChkLv1_1_compare/1

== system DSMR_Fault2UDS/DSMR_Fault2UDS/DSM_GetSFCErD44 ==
  DFC : Inport  OutDataTypeStr=uint8
  DFC_IsoChkLv1_1 : simulink/Logic and Bit Operations/Bitwise Operator  logicop=AND  UseBitMask=on  BitMask=bin2dec('00011000')  BitMaskRealWorld=Stored Integer
  DFC_IsoChkLv1_1_compare : simulink/Logic and Bit Operations/Compare To Constant  relop===  const=24  OutDataTypeStr=boolean
  y : Outport
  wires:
  DFC_IsoChkLv1_1_compare/1 -> y/1
  DFC/1 -> DFC_IsoChkLv1_1/1
  DFC_IsoChkLv1_1/1 -> DFC_IsoChkLv1_1_compare/1

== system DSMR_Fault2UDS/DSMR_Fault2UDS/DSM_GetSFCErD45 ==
  DFC : Inport  OutDataTypeStr=uint8
  DFC_IsoChkLv1_1 : simulink/Logic and Bit Operations/Bitwise Operator  logicop=AND  UseBitMask=on  BitMask=bin2dec('00011000')  BitMaskRealWorld=Stored Integer
  DFC_IsoChkLv1_1_compare : simulink/Logic and Bit Operations/Compare To Constant  relop===  const=24  OutDataTypeStr=boolean
  y : Outport
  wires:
  DFC_IsoChkLv1_1_compare/1 -> y/1
  DFC/1 -> DFC_IsoChkLv1_1/1
  DFC_IsoChkLv1_1/1 -> DFC_IsoChkLv1_1_compare/1

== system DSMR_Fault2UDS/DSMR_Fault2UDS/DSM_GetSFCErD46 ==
  DFC : Inport  OutDataTypeStr=uint8
  DFC_IsoChkLv1_1 : simulink/Logic and Bit Operations/Bitwise Operator  logicop=AND  UseBitMask=on  BitMask=bin2dec('00011000')  BitMaskRealWorld=Stored Integer
  DFC_IsoChkLv1_1_compare : simulink/Logic and Bit Operations/Compare To Constant  relop===  const=24  OutDataTypeStr=boolean
  y : Outport
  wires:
  DFC_IsoChkLv1_1_compare/1 -> y/1
  DFC/1 -> DFC_IsoChkLv1_1/1
  DFC_IsoChkLv1_1/1 -> DFC_IsoChkLv1_1_compare/1

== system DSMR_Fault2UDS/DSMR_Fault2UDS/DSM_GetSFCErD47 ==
  DFC : Inport  OutDataTypeStr=uint8
  DFC_IsoChkLv1_1 : simulink/Logic and Bit Operations/Bitwise Operator  logicop=AND  UseBitMask=on  BitMask=bin2dec('00011000')  BitMaskRealWorld=Stored Integer
  DFC_IsoChkLv1_1_compare : simulink/Logic and Bit Operations/Compare To Constant  relop===  const=24  OutDataTypeStr=boolean
  y : Outport
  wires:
  DFC_IsoChkLv1_1_compare/1 -> y/1
  DFC/1 -> DFC_IsoChkLv1_1/1
  DFC_IsoChkLv1_1/1 -> DFC_IsoChkLv1_1_compare/1

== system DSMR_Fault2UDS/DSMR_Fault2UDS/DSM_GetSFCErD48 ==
  DFC : Inport  OutDataTypeStr=uint8
  DFC_IsoChkLv1_1 : simulink/Logic and Bit Operations/Bitwise Operator  logicop=AND  UseBitMask=on  BitMask=bin2dec('00011000')  BitMaskRealWorld=Stored Integer
  DFC_IsoChkLv1_1_compare : simulink/Logic and Bit Operations/Compare To Constant  relop===  const=24  OutDataTypeStr=boolean
  y : Outport
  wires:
  DFC_IsoChkLv1_1_compare/1 -> y/1
  DFC/1 -> DFC_IsoChkLv1_1/1
  DFC_IsoChkLv1_1/1 -> DFC_IsoChkLv1_1_compare/1

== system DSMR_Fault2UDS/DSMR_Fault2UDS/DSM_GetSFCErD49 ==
  DFC : Inport  OutDataTypeStr=uint8
  DFC_IsoChkLv1_1 : simulink/Logic and Bit Operations/Bitwise Operator  logicop=AND  UseBitMask=on  BitMask=bin2dec('00011000')  BitMaskRealWorld=Stored Integer
  DFC_IsoChkLv1_1_compare : simulink/Logic and Bit Operations/Compare To Constant  relop===  const=24  OutDataTypeStr=boolean
  y : Outport
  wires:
  DFC_IsoChkLv1_1_compare/1 -> y/1
  DFC/1 -> DFC_IsoChkLv1_1/1
  DFC_IsoChkLv1_1/1 -> DFC_IsoChkLv1_1_compare/1

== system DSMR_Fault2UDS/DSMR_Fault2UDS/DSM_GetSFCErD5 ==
  DFC : Inport  OutDataTypeStr=uint8
  DFC_IsoChkLv1_1 : simulink/Logic and Bit Operations/Bitwise Operator  logicop=AND  UseBitMask=on  BitMask=bin2dec('00011000')  BitMaskRealWorld=Stored Integer
  DFC_IsoChkLv1_1_compare : simulink/Logic and Bit Operations/Compare To Constant  relop===  const=24  OutDataTypeStr=boolean
  y : Outport
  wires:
  DFC_IsoChkLv1_1_compare/1 -> y/1
  DFC/1 -> DFC_IsoChkLv1_1/1
  DFC_IsoChkLv1_1/1 -> DFC_IsoChkLv1_1_compare/1

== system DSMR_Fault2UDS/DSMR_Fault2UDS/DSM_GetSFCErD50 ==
  DFC : Inport  OutDataTypeStr=uint8
  DFC_IsoChkLv1_1 : simulink/Logic and Bit Operations/Bitwise Operator  logicop=AND  UseBitMask=on  BitMask=bin2dec('00011000')  BitMaskRealWorld=Stored Integer
  DFC_IsoChkLv1_1_compare : simulink/Logic and Bit Operations/Compare To Constant  relop===  const=24  OutDataTypeStr=boolean
  y : Outport
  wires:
  DFC_IsoChkLv1_1_compare/1 -> y/1
  DFC/1 -> DFC_IsoChkLv1_1/1
  DFC_IsoChkLv1_1/1 -> DFC_IsoChkLv1_1_compare/1

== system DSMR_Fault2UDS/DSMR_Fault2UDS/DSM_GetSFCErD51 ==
  DFC : Inport  OutDataTypeStr=uint8
  DFC_IsoChkLv1_1 : simulink/Logic and Bit Operations/Bitwise Operator  logicop=AND  UseBitMask=on  BitMask=bin2dec('00011000')  BitMaskRealWorld=Stored Integer
  DFC_IsoChkLv1_1_compare : simulink/Logic and Bit Operations/Compare To Constant  relop===  const=24  OutDataTypeStr=boolean
  y : Outport
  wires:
  DFC_IsoChkLv1_1_compare/1 -> y/1
  DFC/1 -> DFC_IsoChkLv1_1/1
  DFC_IsoChkLv1_1/1 -> DFC_IsoChkLv1_1_compare/1

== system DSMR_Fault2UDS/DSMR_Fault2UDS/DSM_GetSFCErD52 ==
  DFC : Inport  OutDataTypeStr=uint8
  DFC_IsoChkLv1_1 : simulink/Logic and Bit Operations/Bitwise Operator  logicop=AND  UseBitMask=on  BitMask=bin2dec('00011000')  BitMaskRealWorld=Stored Integer
  DFC_IsoChkLv1_1_compare : simulink/Logic and Bit Operations/Compare To Constant  relop===  const=24  OutDataTypeStr=boolean
  y : Outport
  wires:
  DFC_IsoChkLv1_1_compare/1 -> y/1
  DFC/1 -> DFC_IsoChkLv1_1/1
  DFC_IsoChkLv1_1/1 -> DFC_IsoChkLv1_1_compare/1

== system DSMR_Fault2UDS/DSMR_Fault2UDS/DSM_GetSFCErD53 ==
  DFC : Inport  OutDataTypeStr=uint8
  DFC_IsoChkLv1_1 : simulink/Logic and Bit Operations/Bitwise Operator  logicop=AND  UseBitMask=on  BitMask=bin2dec('00011000')  BitMaskRealWorld=Stored Integer
  DFC_IsoChkLv1_1_compare : simulink/Logic and Bit Operations/Compare To Constant  relop===  const=24  OutDataTypeStr=boolean
  y : Outport
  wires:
  DFC_IsoChkLv1_1_compare/1 -> y/1
  DFC/1 -> DFC_IsoChkLv1_1/1
  DFC_IsoChkLv1_1/1 -> DFC_IsoChkLv1_1_compare/1

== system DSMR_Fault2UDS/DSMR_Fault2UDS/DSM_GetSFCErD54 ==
  DFC : Inport  OutDataTypeStr=uint8
  DFC_IsoChkLv1_1 : simulink/Logic and Bit Operations/Bitwise Operator  logicop=AND  UseBitMask=on  BitMask=bin2dec('00011000')  BitMaskRealWorld=Stored Integer
  DFC_IsoChkLv1_1_compare : simulink/Logic and Bit Operations/Compare To Constant  relop===  const=24  OutDataTypeStr=boolean
  y : Outport
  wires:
  DFC_IsoChkLv1_1_compare/1 -> y/1
  DFC/1 -> DFC_IsoChkLv1_1/1
  DFC_IsoChkLv1_1/1 -> DFC_IsoChkLv1_1_compare/1

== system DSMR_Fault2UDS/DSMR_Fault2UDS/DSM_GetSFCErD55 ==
  DFC : Inport  OutDataTypeStr=uint8
  DFC_IsoChkLv1_1 : simulink/Logic and Bit Operations/Bitwise Operator  logicop=AND  UseBitMask=on  BitMask=bin2dec('00011000')  BitMaskRealWorld=Stored Integer
  DFC_IsoChkLv1_1_compare : simulink/Logic and Bit Operations/Compare To Constant  relop===  const=24  OutDataTypeStr=boolean
  y : Outport
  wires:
  DFC_IsoChkLv1_1_compare/1 -> y/1
  DFC/1 -> DFC_IsoChkLv1_1/1
  DFC_IsoChkLv1_1/1 -> DFC_IsoChkLv1_1_compare/1

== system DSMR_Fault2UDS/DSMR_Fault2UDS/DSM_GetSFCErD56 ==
  DFC : Inport  OutDataTypeStr=uint8
  DFC_IsoChkLv1_1 : simulink/Logic and Bit Operations/Bitwise Operator  logicop=AND  UseBitMask=on  BitMask=bin2dec('00011000')  BitMaskRealWorld=Stored Integer
  DFC_IsoChkLv1_1_compare : simulink/Logic and Bit Operations/Compare To Constant  relop===  const=24  OutDataTypeStr=boolean
  y : Outport
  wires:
  DFC_IsoChkLv1_1_compare/1 -> y/1
  DFC/1 -> DFC_IsoChkLv1_1/1
  DFC_IsoChkLv1_1/1 -> DFC_IsoChkLv1_1_compare/1

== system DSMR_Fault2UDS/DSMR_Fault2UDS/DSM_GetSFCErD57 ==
  DFC : Inport  OutDataTypeStr=uint8
  DFC_IsoChkLv1_1 : simulink/Logic and Bit Operations/Bitwise Operator  logicop=AND  UseBitMask=on  BitMask=bin2dec('00011000')  BitMaskRealWorld=Stored Integer
  DFC_IsoChkLv1_1_compare : simulink/Logic and Bit Operations/Compare To Constant  relop===  const=24  OutDataTypeStr=boolean
  y : Outport
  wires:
  DFC_IsoChkLv1_1_compare/1 -> y/1
  DFC/1 -> DFC_IsoChkLv1_1/1
  DFC_IsoChkLv1_1/1 -> DFC_IsoChkLv1_1_compare/1

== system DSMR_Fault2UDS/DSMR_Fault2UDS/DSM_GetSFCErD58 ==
  DFC : Inport  OutDataTypeStr=uint8
  DFC_IsoChkLv1_1 : simulink/Logic and Bit Operations/Bitwise Operator  logicop=AND  UseBitMask=on  BitMask=bin2dec('00011000')  BitMaskRealWorld=Stored Integer
  DFC_IsoChkLv1_1_compare : simulink/Logic and Bit Operations/Compare To Constant  relop===  const=24  OutDataTypeStr=boolean
  y : Outport
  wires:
  DFC_IsoChkLv1_1_compare/1 -> y/1
  DFC/1 -> DFC_IsoChkLv1_1/1
  DFC_IsoChkLv1_1/1 -> DFC_IsoChkLv1_1_compare/1

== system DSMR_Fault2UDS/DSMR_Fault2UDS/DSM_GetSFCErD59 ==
  DFC : Inport  OutDataTypeStr=uint8
  DFC_IsoChkLv1_1 : simulink/Logic and Bit Operations/Bitwise Operator  logicop=AND  UseBitMask=on  BitMask=bin2dec('00011000')  BitMaskRealWorld=Stored Integer
  DFC_IsoChkLv1_1_compare : simulink/Logic and Bit Operations/Compare To Constant  relop===  const=24  OutDataTypeStr=boolean
  y : Outport
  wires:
  DFC_IsoChkLv1_1_compare/1 -> y/1
  DFC/1 -> DFC_IsoChkLv1_1/1
  DFC_IsoChkLv1_1/1 -> DFC_IsoChkLv1_1_compare/1

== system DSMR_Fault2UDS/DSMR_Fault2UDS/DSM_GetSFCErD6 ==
  DFC : Inport  OutDataTypeStr=uint8
  DFC_IsoChkLv1_1 : simulink/Logic and Bit Operations/Bitwise Operator  logicop=AND  UseBitMask=on  BitMask=bin2dec('00011000')  BitMaskRealWorld=Stored Integer
  DFC_IsoChkLv1_1_compare : simulink/Logic and Bit Operations/Compare To Constant  relop===  const=24  OutDataTypeStr=boolean
  y : Outport
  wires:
  DFC_IsoChkLv1_1_compare/1 -> y/1
  DFC/1 -> DFC_IsoChkLv1_1/1
  DFC_IsoChkLv1_1/1 -> DFC_IsoChkLv1_1_compare/1

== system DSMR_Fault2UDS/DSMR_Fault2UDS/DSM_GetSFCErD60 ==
  DFC : Inport  OutDataTypeStr=uint8
  DFC_IsoChkLv1_1 : simulink/Logic and Bit Operations/Bitwise Operator  logicop=AND  UseBitMask=on  BitMask=bin2dec('00011000')  BitMaskRealWorld=Stored Integer
  DFC_IsoChkLv1_1_compare : simulink/Logic and Bit Operations/Compare To Constant  relop===  const=24  OutDataTypeStr=boolean
  y : Outport
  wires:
  DFC_IsoChkLv1_1_compare/1 -> y/1
  DFC/1 -> DFC_IsoChkLv1_1/1
  DFC_IsoChkLv1_1/1 -> DFC_IsoChkLv1_1_compare/1

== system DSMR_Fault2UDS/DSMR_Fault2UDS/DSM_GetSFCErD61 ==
  DFC : Inport  OutDataTypeStr=uint8
  DFC_IsoChkLv1_1 : simulink/Logic and Bit Operations/Bitwise Operator  logicop=AND  UseBitMask=on  BitMask=bin2dec('00011000')  BitMaskRealWorld=Stored Integer
  DFC_IsoChkLv1_1_compare : simulink/Logic and Bit Operations/Compare To Constant  relop===  const=24  OutDataTypeStr=boolean
  y : Outport
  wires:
  DFC_IsoChkLv1_1_compare/1 -> y/1
  DFC/1 -> DFC_IsoChkLv1_1/1
  DFC_IsoChkLv1_1/1 -> DFC_IsoChkLv1_1_compare/1

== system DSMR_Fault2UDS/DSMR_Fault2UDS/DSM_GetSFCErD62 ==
  DFC : Inport  OutDataTypeStr=uint8
  DFC_IsoChkLv1_1 : simulink/Logic and Bit Operations/Bitwise Operator  logicop=AND  UseBitMask=on  BitMask=bin2dec('00011000')  BitMaskRealWorld=Stored Integer
  DFC_IsoChkLv1_1_compare : simulink/Logic and Bit Operations/Compare To Constant  relop===  const=24  OutDataTypeStr=boolean
  y : Outport
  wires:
  DFC_IsoChkLv1_1_compare/1 -> y/1
  DFC/1 -> DFC_IsoChkLv1_1/1
  DFC_IsoChkLv1_1/1 -> DFC_IsoChkLv1_1_compare/1

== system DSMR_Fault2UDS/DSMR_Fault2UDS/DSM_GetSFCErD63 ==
  DFC : Inport  OutDataTypeStr=uint8
  DFC_IsoChkLv1_1 : simulink/Logic and Bit Operations/Bitwise Operator  logicop=AND  UseBitMask=on  BitMask=bin2dec('00011000')  BitMaskRealWorld=Stored Integer
  DFC_IsoChkLv1_1_compare : simulink/Logic and Bit Operations/Compare To Constant  relop===  const=24  OutDataTypeStr=boolean
  y : Outport
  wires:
  DFC_IsoChkLv1_1_compare/1 -> y/1
  DFC/1 -> DFC_IsoChkLv1_1/1
  DFC_IsoChkLv1_1/1 -> DFC_IsoChkLv1_1_compare/1
